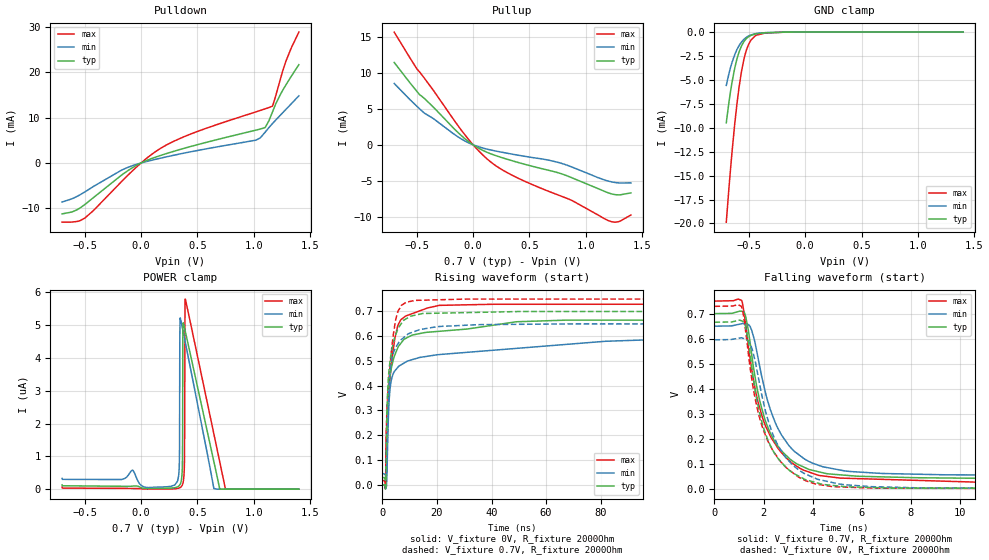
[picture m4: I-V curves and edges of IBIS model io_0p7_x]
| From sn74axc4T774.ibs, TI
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|   io_0p7_x Model
[Model]   io_0p7_x
Model_type   I/O
Polarity   Non-Inverting
Enable   Active-Low
Vinl = 0.21
Vinh = 0.49
Vmeas = 0.35
Vref = 0
Cref = 2pF
Rref = 100000
|   typ   min   max
C_comp   1.852pF   1.651pF   2.136pF
[Model spec]
|subparameter
Vinl   0.21   0.195   0.225
Vinh   0.49   0.455   0.525
| Where Nom  PVT is Nominal Process, 0.7V, 27C
|   Fast PVT is Strong Process,  0.75V, -40C
|   Slow PVT is Weak Process,   0.65V, 130C
[Voltage Range]   0.7   0.65   0.75
|Junction Temperature
[Temperature Range]   27   130   -40
[Pullup Reference]   0.7   0.65   0.75
[Pulldown Reference]   0   -0   -0
[Power Clamp Reference]   0.7   0.65   0.75
[GND Clamp Reference]   0   0   0
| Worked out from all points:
|   slope of the pulldown table from 0 to 0.105 V, typ, clamps not added: 97 ohm
|   slope of the pullup table from 0 to 0.105 V, typ, clamps not added: 115 ohm
|   GND clamp passes 1 mA (typ) near -0.54 V on its own axis
|   falling waveform, V_fixture 0.7V, R_fixture 2000Ohm: 20-80 % time 1.17ns typ, 1.34ns min, 1.25ns max; typ from 0.7 V to 0.029 V
|   rising waveform, V_fixture 0V, R_fixture 2000Ohm: 20-80 % time 3.37ns typ, 4.02ns min, 3.11ns max; typ from 0 V to 0.666 V
|   rising waveform, V_fixture 0.7V, R_fixture 2000Ohm: 20-80 % time 2.36ns typ, 2.16ns min, 2.61ns max; typ from 0.029 V to 0.7 V
|   falling waveform, V_fixture 0V, R_fixture 2000Ohm: 20-80 % time 1.06ns typ, 1.24ns min, 1.1ns max; typ from 0.666 V to 0 V
[Pulldown]
|   Voltage   I(typ)   I(min)   I(max)
-700mV    -11.24mA   -8.62mA    -13.07mA
-613.9mV  -10.82mA   -7.924mA   -13.04mA
-496.3mV  -9.135mA   -6.354mA   -12.12mA
-86.8mV   -1.205mA   -684.4uA   -1.987mA
85.4mV    904uA      551.5uA    1.733mA
219.8mV   2.037mA    1.327mA    3.904mA
501.2mV   4.053mA    2.765mA    6.975mA
1.02V     7.267mA    5.047mA    11.3mA
1.1V      7.82mA     6.754mA    11.95mA
1.165V    11.18mA    8.677mA    12.54mA
1.282V    17.14mA    11.76mA    22.29mA
1.4V      21.71mA    14.83mA    28.91mA
[GND Clamp]
|   Voltage   I(typ)   I(min)   I(max)
-700mV    -9.473mA   -5.569mA   -19.87mA
-674.8mV  -7.198mA   -4.264mA   -16.07mA
-649.6mV  -5.285mA   -3.192mA   -12.61mA
-622.3mV  -3.629mA   -2.276mA   -9.304mA
-584.5mV  -2.013mA   -1.371mA   -5.599mA
-544.6mV  -1.015mA   -772.1uA   -2.899mA
-521.5mV  -677.6uA   -547uA     -1.878mA
-481.6mV  -348uA     -300.8uA   -843.7uA
-443.8mV  -200.2uA   -174.6uA   -401uA
-351.4mV  -69.33uA   -55.44uA   -97.88uA
-175mV    -6.308uA   -6.304uA   -6.326uA
1.4V      0A         0A         0A
[Pullup]
|   Voltage   I(typ)   I(min)   I(max)
-700mV    11.42mA    8.504mA    15.64mA
-500.5mV  7.445mA    5.37mA     10.57mA
-433.3mV  6.439mA    4.402mA    9.258mA
-145.6mV  1.877mA    1.221mA    2.904mA
-2.8mV    28.63uA    16.85uA    49.69uA
158.9mV   -1.264mA   -726uA     -2.416mA
413mV     -2.512mA   -1.479mA   -4.735mA
765.8mV   -3.931mA   -2.49mA    -7.031mA
881.3mV   -4.609mA   -3.111mA   -7.761mA
1.2V      -6.673mA   -5.042mA   -10.52mA
1.291V    -6.947mA   -5.286mA   -10.66mA
1.4V      -6.671mA   -5.282mA   -9.735mA
[POWER Clamp]
|   Voltage   I(typ)   I(min)   I(max)
-700mV    133.1nA    328.5nA    61.75nA
301.7mV   46.57nA    137.1nA    11.39nA
337.4mV   102.3nA    571.4nA    34.33nA
341.6mV   118.7nA    1.205uA    40.18nA
345.8mV   140.3nA    5.17uA     47.41nA
362.6mV   405.2nA    4.989uA    104.1nA
368.9mV   1.503uA    4.883uA    151.5nA
371mV     4.89uA     4.848uA    174.5nA
385.7mV   4.915uA    4.597uA    910.3nA
392mV     4.819uA    4.489uA    5.794uA
751.1mV   0A         0A         0A
1.4V      0A         0A         0A
[Ramp]
R_load = 2000
|   typ   min   max
dV/dt_r   0.399437/3.28355e-09   0.357403/3.95108e-09   0.437449/3.09277e-09
dV/dt_f   0.402409/1.16614e-09   0.362784/1.33847e-09   0.439744/1.24446e-09
[Falling Waveform]
V_fixture = 0.7V
V_fixture_min = 0.65V
V_fixture_max = 0.75V
R_fixture = 2000Ohm
C_fixture = 0F
|   Time   V(typ)   V(min)   V(max)
0s        700mV      650mV      750mV
1.111ns   709.4mV    659.7mV    753.1mV
1.223ns   703.4mV    660mV      693.4mV
1.521ns   535.7mV    633.2mV    477.5mV
2.033ns   286mV      405mV      264.8mV
2.599ns   170.1mV    240.2mV    162mV
3.49ns    94.94mV    133.7mV    83.05mV
5.516ns   54.09mV    70.58mV    43.03mV
13.28ns   41.2mV     55.85mV    20.44mV
500ns     29.31mV    45.33mV    17.09mV
[Rising Waveform]
V_fixture = 0V
V_fixture_min = 0V
V_fixture_max = 0V
R_fixture = 2000Ohm
C_fixture = 0F
|   Time   V(typ)   V(min)   V(max)
0s        504.7nV    3.721uV    113nV
1.249ns   -9.806mV   -16.23mV   39.57mV
1.545ns   157.4mV    1.23mV     231.8mV
1.888ns   317.2mV    141.5mV    308.1mV
2.438ns   408.3mV    329.1mV    385.4mV
3.535ns   482.8mV    434.1mV    506.4mV
5.553ns   550.5mV    472.5mV    638.2mV
20.75ns   619.7mV    525.6mV    724.3mV
115.3ns   664.8mV    592mV      729mV
500ns     665.7mV    595.7mV    729.1mV
[Rising Waveform]
V_fixture = 0.7V
V_fixture_min = 0.65V
V_fixture_max = 0.75V
R_fixture = 2000Ohm
C_fixture = 0F
|   Time   V(typ)   V(min)   V(max)
0s        29.31mV    45.33mV    17.09mV
1.116ns   13.07mV    37.56mV    5.741mV
1.289ns   31.02mV    32.48mV    90.78mV
1.481ns   146mV      41.4mV     231.3mV
1.888ns   365.9mV    201.9mV    345.1mV
2.599ns   479.3mV    428.7mV    452.9mV
4.727ns   600.5mV    551.3mV    656.8mV
6.928ns   651.1mV    586.2mV    723.9mV
11.93ns   684.7mV    619.5mV    744.6mV
500ns     700mV      650mV      750mV
[Falling Waveform]
|Gnd
V_fixture = 0V
V_fixture_min = 0V
V_fixture_max = 0V
R_fixture = 2000Ohm
C_fixture = 0F
|   Time   V(typ)   V(min)   V(max)
0s        665.7mV    595.7mV    729.1mV
1.106ns   671.3mV    603.7mV    728.3mV
1.301ns   633.6mV    596.9mV    608.3mV
1.542ns   472.8mV    557.2mV    426.2mV
1.787ns   327.6mV    447.3mV    304.1mV
2.216ns   187.8mV    264.7mV    183.8mV
2.707ns   109.6mV    155.9mV    108.9mV
4.207ns   24.39mV    39.29mV    19.29mV
6.512ns   6.301mV    9.729mV    4.141mV
500ns     466.3nV    3.722uV    130.9nV
